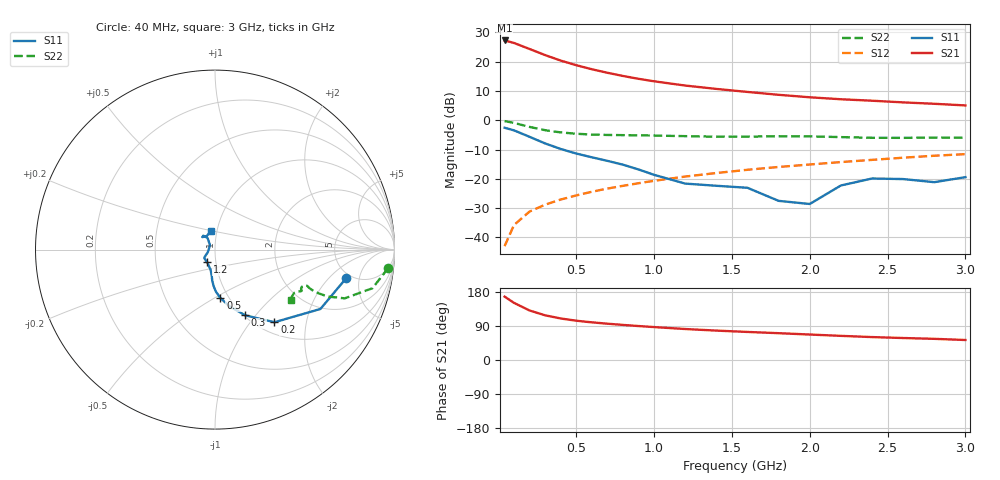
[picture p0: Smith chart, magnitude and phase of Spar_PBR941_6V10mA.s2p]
! Filename:  PBR941N.S2P  Version:  3.0
! NXP part #:  PBR941  Date: July 1998
! Bias condition:  Vce=6V, Ic=10mA
#  MHz  S  MA  R 50
! Freq  S11  S21  S12  S22
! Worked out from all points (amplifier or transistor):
!   21 points, 40 MHz to 3 GHz, reference 50 ohm
!   highest |S21| = 27.3 dB at 40 MHz (marker M1)
!   |S21| within 3 dB of that: start of sweep to 204.5 MHz
!   unconditionally stable (mu >= 1): 1.012 GHz to 2.351 GHz
!   at 300 MHz: K = 0.69, MSG = 25.5 dB, |S12| = -28.8 dB
!   at 1 GHz: K = 1.00, MSG = 17.0 dB, |S12| = -20.7 dB
!   at 3 GHz: K = 0.98, MSG = 8.3 dB, |S12| = -11.5 dB
!   lowest NFmin = 1.70 dB at 500 MHz
!   S11 on the Smith chart (normalised r, x): 40 MHz: 4.47, -3.25; 200 MHz: 1.19, -1.32; 300 MHz: 1.01, -0.89; 500 MHz: 0.91, -0.53; 1.2 GHz: 0.91, -0.13; 3 GHz: 0.94, +0.20
40  0.7473 -12.4  23.1 167.3  0.007101 83.6  0.97 -6.1
100  0.6742 -29.4  20.94 150.8  0.01628 76.7  0.9035 -13.8
200  0.523 -50.7  16.53 130.7  0.02766 70.6  0.7722 -20.6
300  0.4034 -65.3  13 118.0  0.03628 69.8  0.6786 -22.6
400  0.3246 -75.9  10.48 109.6  0.0444 70.4  0.622 -22.9
500  0.2711 -83.7  8.734 103.7  0.05219 71.8  0.5898 -22.7
600  0.2338 -88.8  7.452 99.4  0.06028 72.9  0.5717 -22.3
700  0.2033 -92.2  6.484 95.8  0.06831 74.2  0.5626 -22.0
800  0.1748 -95.0  5.723 92.6  0.07613 74.9  0.5584 -21.7
900  0.1451 -97.4  5.115 89.6  0.08429 75.5  0.5538 -21.6
1000  0.1173 -101.8  4.637 86.9  0.09269 75.7  0.5488 -21.5
1200  0.08316 -121.2  3.924 81.8  0.1096 76.4  0.5368 -22.0
1400  0.07628 -141.0  3.437 77.6  0.126 76.4  0.5259 -23.3
1600  0.07049 -144.8  3.052 74.0  0.143 76.6  0.5267 -24.6
1800  0.04216 -160.4  2.727 70.8  0.1598 76.8  0.5347 -25.4
2000  0.03729 138.7  2.474 67.2  0.1761 76.3  0.5321 -25.9
2200  0.07714 122.4  2.289 63.7  0.1938 75.4  0.517 -26.7
2400  0.1015 130.2  2.161 60.5  0.2112 75.0  0.5031 -28.6
2600  0.09933 135.4  2.024 58.0  0.23 74.6  0.5016 -31.3
2800  0.08785 123.8  1.916 55.9  0.2485 74.2  0.5085 -33.1
3000  0.1071 100.9  1.796 52.8  0.2647 73.2  0.5049 -33.5
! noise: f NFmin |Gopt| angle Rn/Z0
500  1.702  0.176  2.23  0.345
900  1.72  0.165  18.62  0.237
1000  1.76  0.172  29.24  0.258
2000  2.331  0.065  -139.9  0.254
